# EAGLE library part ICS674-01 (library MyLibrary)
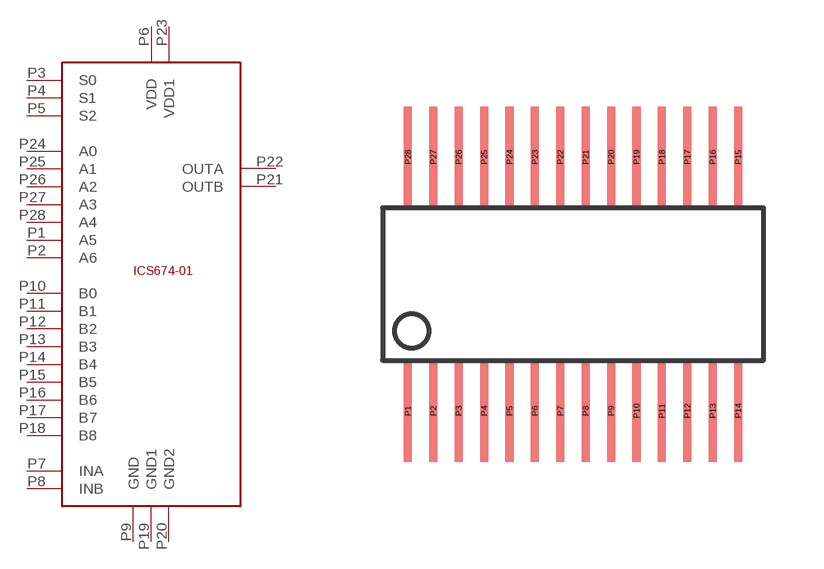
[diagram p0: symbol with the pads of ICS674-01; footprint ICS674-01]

Designator prefix -

## ICS674-01  [ICS674-01]
P1  A5
P2  A6
P3  S0
P4  S1
P5  S2
P6  VDD
P7  INA
P8  INB
P9  GND
P10  B0
P11  B1
P12  B2
P13  B3
P14  B4
P15  B5
P16  B6
P17  B7
P18  B8
P19  GND1
P20  GND2
P21  OUTB
P22  OUTA
P23  VDD1
P24  A0
P25  A1
P26  A2
P27  A3
P28  A4

## Footprint ICS674-01 (pad centres in mm)
smd 0.203 x 2.54: P1 -4.445,-3.175; P2 -3.81,-3.175; P3 -3.175,-3.175; P4 -2.54,-3.175; P5 -1.905,-3.175; P6 -1.27,-3.175; P7 -0.635,-3.175; P8 0,-3.175; P9 0.635,-3.175; P10 1.27,-3.175; P11 1.905,-3.175; P12 2.54,-3.175; P13 3.175,-3.175; P14 3.81,-3.175; P15 3.81,3.175; P16 3.175,3.175; P17 2.54,3.175; P18 1.905,3.175; P19 1.27,3.175; P20 0.635,3.175; P21 0,3.175; P22 -0.635,3.175; P23 -1.27,3.175; P24 -1.905,3.175; P25 -2.54,3.175; P26 -3.175,3.175; P27 -3.81,3.175; P28 -4.445,3.175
